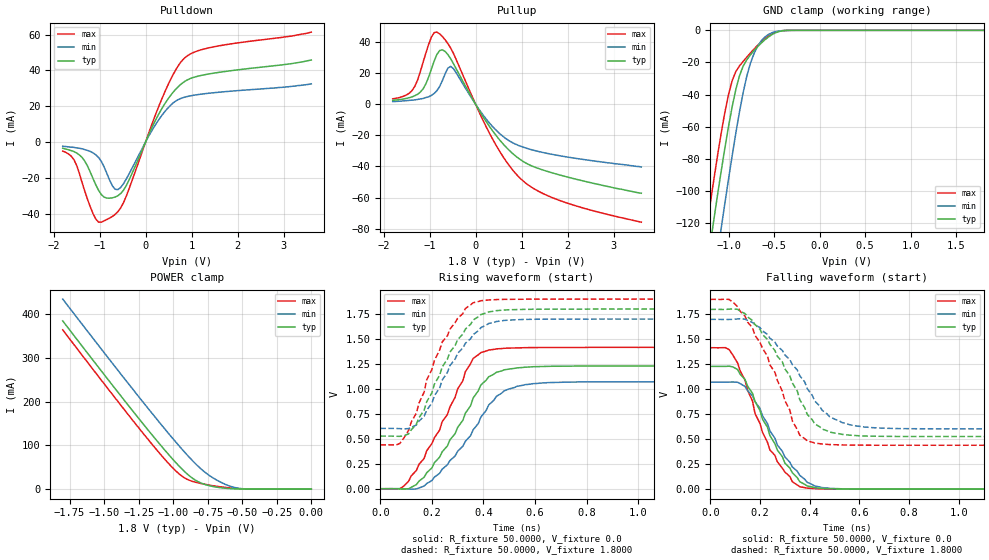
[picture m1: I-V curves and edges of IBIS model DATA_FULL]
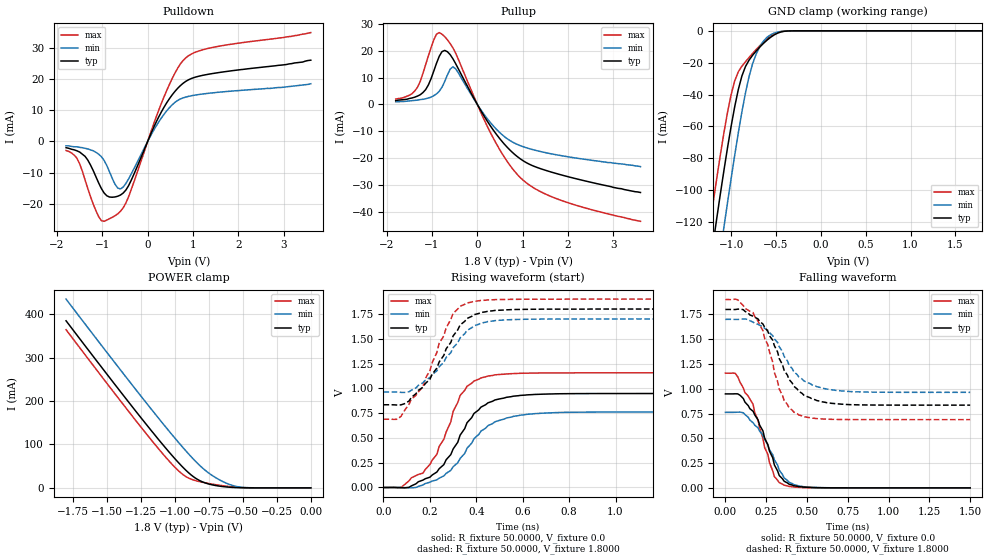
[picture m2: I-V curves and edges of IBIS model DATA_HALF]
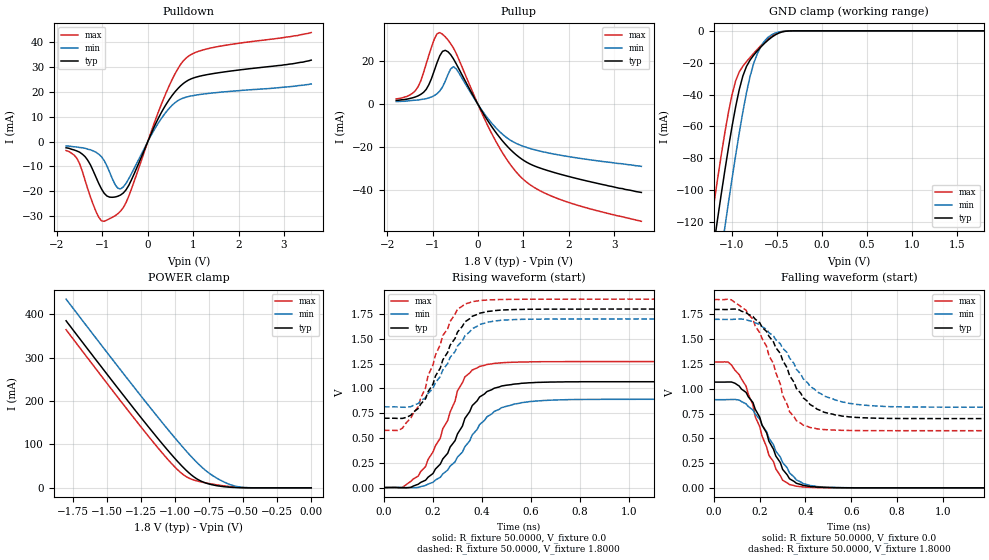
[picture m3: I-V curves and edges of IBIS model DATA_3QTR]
| IBIS file usesk1g16ai.ibs created by s2ibis3 verion 1.1
| North Carolina State University, ERL, 2006
| This Model is valid for Industrial Temperature Range -40C<=Tc<=85C
| Valid for LPDDR-333/400 operation
| Part Number   VDD/VDDQ   Package   Architecture
| SCE18K1G160AF   1.8 +0.1/-0.1  60-Ball FBGA   64Meg x 16
[IBIS Ver]   3.2
[File name]  usesk1g16ai.ibs
[File Rev]   1.2
[Date]   2015-10-27
[Source]   Simulation of a silicon level SPICE model
[Notes]   IBIS Characteristics for I/O Buffer
   IBIS Model Revision History:
Rev 1.1: 2015-10-27
   - IBIS model file initial creation
Rev 1.2: 2016-10-27
   - Updata company and other informations
[disclaimer] The IBIS models are for modeling purpose only and are
   subject to change without any notice. UniIC is not
   responsible for any problems the models may cause.
[Copyright]  Copyright 2015 UniIC Semiconductors Corp. All rights reserved
|   Component SCE18K1G160AF
[Component]   SCE18K1G160AF
[Manufacturer]  UniIC Semiconductors Corp.
| All balls excluding NC, POWER and GND (R[Ohm], L[H], C[F])
[Package]   | 60-Ball FBGA
|Variable   typ   min   max
R_pkg   366m   250m   672m
L_pkg   1.68n   1.12n   2.83n
C_pkg   0.31p   0.20p   0.55p
[Pin]   signal_name model_name   R_pin   L_pin   C_pin
A1   VSS   GND
A2   DQ15   DQ   374m   1.51n   0.32p
A3   VSSQ   GND
A7   VDDQ   POWER
A8   DQ0   DQ   390m   1.48n   0.35p
A9   VDD   POWER
B2   DQ13   DQ   444m   2n   0.4p
B3   DQ14   DQ   332m   1.35n   0.29p
B7   DQ1   DQ   268m   1.19n   0.25p
B8   DQ2   DQ   410m   1.6n   0.37p
B9   VSSQ   GND
C1   VSSQ   GND
C2   DQ11   DQ   370m   1.5n   0.34p
C3   DQ12   DQ   318m   1.58n   0.29p
C7   DQ3   DQ   294m   1.27n   0.28p
C8   DQ4   DQ   387m   1.66n   0.36p
C9   VDDQ   POWER
D1   VDDQ   POWER
D2   DQ9   DQ   391m   1.83n   0.33p
D3   DQ10   DQ   267m   1.14n   0.24p
D7   DQ5   DQ   250m   1.12n   0.27p
D8   DQ6   DQ   405m   1.87n   0.32p
D9   VSSQ   GND
E1   VSSQ   GND
E2   UDQS   DQ   406m   1.72n   0.37p
E3   DQ8   DQ   276m   1.28n   0.25p
E7   DQ7   DQ   275m   1.47n   0.21p
E8   LDQS   DQ   395m   1.59n   0.32p
E9   VDDQ   POWER
F1   VSS   GND
F2   UDM   DATA_RCV   388m   1.82n   0.32p
F7   A13   CLKCA_RCV   264m   1.18n   0.24p
F8   LDM   DATA_RCV   398m   1.54n   0.36p
F9   VDD   POWER
G1   CKE   CLKCA_RCV   453m   2.62n   0.36p
G2   CK   CLKCA_RCV   364m   1.97n   0.32p
G3   CK#   CLKCA_RCV   353m   1.72n   0.25p
G7   WE#   CLKCA_RCV   284m   1.32n   0.26p
G8   CAS#   CLKCA_RCV   381m   1.69n   0.35p
G9   RAS#   CLKCA_RCV   474m   2.32n   0.4p
H1   A9   CLKCA_RCV   457m   2.73n   0.33p
H2   A11   CLKCA_RCV   388m   2.17n   0.29p
H3   A12   CLKCA_RCV   263m   1.36n   0.25p
H7   CS#   CLKCA_RCV   262m   1.22n   0.24p
H8   BA0   CLKCA_RCV   394m   1.67n   0.36p
H9   BA1   CLKCA_RCV   508m   2.19n   0.42p
J1   A6   CLKCA_RCV   672m   2.79n   0.55p
J2   A7   CLKCA_RCV   380m   1.64n   0.3p
J3   A8   CLKCA_RCV   253m   1.34n   0.2p
J7   A10   CLKCA_RCV   263m   1.28n   0.22p
J8   A0   CLKCA_RCV   364m   1.68n   0.29p
J9   A1   CLKCA_RCV   661m   2.83n   0.54p
K1   VSS   GND
K2   A4   CLKCA_RCV   412m   1.87n   0.34p
K3   A5   CLKCA_RCV   266m   1.3n   0.23p
K7   A2   CLKCA_RCV   250m   1.18n   0.24p
K8   A3   CLKCA_RCV   367m   1.75n   0.31p
K9   VDD   POWER
|*****************************  Diff Pin  *************************************
[Diff Pin]  inv_pin  vdiff   tdelay_typ  tdelay_min  tdelay_max
G2   G3   1.08V   NA   NA   NA
|*****************************  Model Selector ********************************
[Model Selector]   DQ
DATA_FULL   Full-Strength Output Driver
DATA_3QTR   75% Strength Output Driver
DATA_HALF   Half-Strength Output Driver
DATA_RCV   Data/Data Strobe/Data Mask Receiver
| Models and submodels in the file (5): DATA_FULL (I/O), DATA_HALF (I/O), DATA_3QTR (I/O), DATA_RCV (Input), CLKCA_RCV (Input)
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|   Model DATA_FULL
[Model]  DATA_FULL
Model_type   I/O
Polarity   Non-Inverting
Enable   Active-High
Vinl  = 360.000mV
Vinh  = 1440.000mV
Vmeas = 900.000mV
Cref  = 20.000pF
C_comp   2.0990pF   2.0750pF   2.3110pF
[Temperature Range]   25.0000   85.0000   -40.0000
[Voltage Range]   1.8000V   1.7000V   1.9000V
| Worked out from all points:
|   slope of the pulldown table from 0 to 0.27 V, typ, clamps not added: 18.2 ohm
|   slope of the pullup table from 0 to 0.27 V, typ, clamps not added: 21 ohm
|   GND clamp passes 1 mA (typ) near -0.46 V on its own axis
|   POWER clamp passes 1 mA (typ) near -0.57 V on its own axis
|   rising waveform, R_fixture 50.0000, V_fixture 0.0: 20-80 % time 173ps typ, 179ps min, 163ps max; typ from 0 V to 1.23 V
|   rising waveform, R_fixture 50.0000, V_fixture 1.8000: 20-80 % time 150ps typ, 150ps min, 139ps max; typ from 0.527 V to 1.8 V
|   falling waveform, R_fixture 50.0000, V_fixture 0.0: 20-80 % time 143ps typ, 148ps min, 137ps max; typ from 1.23 V to 0 V
|   falling waveform, R_fixture 50.0000, V_fixture 1.8000: 20-80 % time 174ps typ, 187ps min, 155ps max; typ from 1.8 V to 0.527 V
[Pulldown]
|Voltage   I(typ)   I(min)   I(max)
-1.8V     -3.5mA     -2.4mA     -5.1mA
-1.56V    -5.3mA     -3mA       -9.7mA
-1.38V    -8.6mA     -3.8mA     -22.6mA
-1.14V    -20.5mA    -6.1mA     -40.14mA
-960mV    -29.42mA   -10.9mA    -44.81mA
-720mV    -31.19mA   -24.52mA   -41.6mA
-600mV    -29.99mA   -26.62mA   -38.88mA
-420mV    -24.42mA   -20.73mA   -30.32mA
300mV     16.25mA    12.96mA    20.78mA
840mV     33.67mA    24.97mA    46.74mA
1.44V     38.29mA    27.41mA    52.96mA
3.6V      45.8mA     32.5mA     61.4mA
[Pullup]
|Voltage   I(typ)   I(min)   I(max)
-1.8V     2.5mA      1.7mA      3.5mA
-1.38V    4.7mA      2.6mA      8.8mA
-1.26V    6.4mA      3.1mA      15.5mA
-1.14V    9.9mA      3.7mA      26.99mA
-960mV    22.59mA    5.67mA     43.09mA
-840mV    31.99mA    8.72mA     46.37mA
-720mV    34.94mA    15.29mA    43.47mA
-540mV    29.17mA    24.33mA    36.08mA
300mV     -14.19mA   -12.02mA   -18.52mA
960mV     -35.32mA   -26.79mA   -47.34mA
1.86V     -45.72mA   -33.27mA   -62.2mA
3.6V      -57.2mA    -40.3mA    -75.8mA
[GND_clamp]
|Voltage   I(typ)   I(min)   I(max)
-1.8V     -382.1mA   -420.9mA   -357.5mA
-1.24V    -149mA     -187mA     -123.6mA
-1.16V    -117.7mA   -154.8mA   -92.62mA
-1.08V    -87.61mA   -123.2mA   -63.92mA
-1V       -59.95mA   -92.78mA   -40.06mA
-960mV    -47.64mA   -78.15mA   -31.42mA
-880mV    -28.39mA   -50.93mA   -22.22mA
-800mV    -18.4mA    -28.71mA   -16.75mA
-680mV    -10.16mA   -9.871mA   -9.318mA
-560mV    -4.068mA   -2.483mA   -3.393mA
-360mV    -77.71uA   -65.53uA   -56.11uA
1.8V      3.312nA    24.23nA    479.4pA
[POWER_clamp]
|Voltage   I(typ)   I(min)   I(max)
-1.8V     384.7mA    434.6mA    364.2mA
-1.38V    213.6mA    263.5mA    192.2mA
-1.16V    126.8mA    176.1mA    105.2mA
-1.02V    74.41mA    122.2mA    54.12mA
-960mV    53.65mA    99.93mA    35.62mA
-920mV    40.93mA    85.55mA    26.2mA
-840mV    20.7mA     58.65mA    16mA
-780mV    11.76mA    41.29mA    11.75mA
-680mV    4.343mA    19.92mA    6.353mA
-580mV    1.115mA    5.926mA    2.488mA
-460mV    97.61uA    425uA      237.2uA
0V        3.312nA    8.237nA    602.9pA
[Ramp]
| variable   typ   min   max
dV/dt_r  0.7374/0.1699n   0.6426/0.1795n   0.8496/0.1636n
dV/dt_f  0.7638/0.1717n   0.6576/0.1866n   0.8762/0.1570n
R_load = 50.0000
[Rising Waveform]
R_fixture= 50.0000
V_fixture= 0.0
V_fixture_min= 0.0
V_fixture_max= 0.0
|time   V(typ)   V(min)   V(max)
0s        0V         0V         0V
90.91ps   -4.216mV   -497.2uV   25.92mV
170ps     115mV      26.85mV    303.9mV
260ps     428mV      239.4mV    743.1mV
330ps     757mV      475.9mV    1.173V
360ps     908.9mV    590.6mV    1.306V
390ps     1.04V      719.2mV    1.364V
480ps     1.191V     980.7mV    1.407V
590ps     1.222V     1.052V     1.414V
1.5ns     1.229V     1.071V     1.416V
[Rising Waveform]
R_fixture= 50.0000
V_fixture= 1.8000
V_fixture_min= 1.7000
V_fixture_max= 1.9000
|time   V(typ)   V(min)   V(max)
0s        527mV      604mV      439.6mV
75.76ps   524.6mV    601.8mV    452.9mV
140ps     646.7mV    638.8mV    758.4mV
180ps     871.9mV    786.2mV    1.091V
200ps     959.8mV    857mV      1.194V
240ps     1.22V      1.089V     1.47V
360ps     1.69V      1.544V     1.863V
420ps     1.771V     1.655V     1.891V
520ps     1.794V     1.692V     1.898V
1.5ns     1.8V       1.7V       1.9V
[Falling Waveform]
R_fixture= 50.0000
V_fixture= 0.0
V_fixture_min= 0.0
V_fixture_max= 0.0
|time   V(typ)   V(min)   V(max)
0s        1.229V     1.071V     1.416V
75.76ps   1.231V     1.072V     1.397V
110ps     1.197V     1.07V      1.262V
170ps     959.1mV    934.7mV    880.3mV
180ps     877.9mV    875.6mV    757.3mV
240ps     535.2mV    582.8mV    392.4mV
300ps     261.6mV    322.9mV    171.5mV
360ps     74.58mV    138.3mV    24.6mV
480ps     4.177mV    8.446mV    1.502mV
1.5ns     0V         -795nV     0V
[Falling Waveform]
R_fixture= 50.0000
V_fixture= 1.8000
V_fixture_min= 1.7000
V_fixture_max= 1.9000
|time   V(typ)   V(min)   V(max)
0s        1.8V       1.7V       1.9V
75.76ps   1.802V     1.699V     1.899V
170ps     1.688V     1.669V     1.615V
260ps     1.388V     1.472V     1.17V
330ps     1.063V     1.247V     684.1mV
360ps     894.7mV    1.136V     540.1mV
390ps     748.2mV    1.006V     483.8mV
480ps     571.5mV    724.7mV    446.4mV
590ps     535.5mV    631.1mV    440.6mV
1.5ns     527mV      604mV      439.6mV
|   Model DATA_HALF
[Model]  DATA_HALF
Model_type   I/O
Polarity   Non-Inverting
Enable   Active-High
Vinl  = 360.000mV
Vinh  = 1440.000mV
Vmeas = 900.000mV
Cref  = 20.000pF
C_comp   2.0990pF   2.0750pF   2.3110pF
[Temperature Range]   25.0000   85.0000   -40.0000
[Voltage Range]   1.8000V   1.7000V   1.9000V
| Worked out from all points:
|   slope of the pulldown table from 0 to 0.27 V, typ, clamps not added: 31.3 ohm
|   slope of the pullup table from 0 to 0.27 V, typ, clamps not added: 36.1 ohm
|   GND clamp passes 1 mA (typ) near -0.46 V on its own axis
|   POWER clamp passes 1 mA (typ) near -0.57 V on its own axis
|   rising waveform, R_fixture 50.0000, V_fixture 0.0: 20-80 % time 156ps typ, 168ps min, 130ps max; typ from 0 V to 0.948 V
|   rising waveform, R_fixture 50.0000, V_fixture 1.8000: 20-80 % time 149ps typ, 150ps min, 141ps max; typ from 0.834 V to 1.8 V
|   falling waveform, R_fixture 50.0000, V_fixture 0.0: 20-80 % time 140ps typ, 145ps min, 136ps max; typ from 0.948 V to 0 V
|   falling waveform, R_fixture 50.0000, V_fixture 1.8000: 20-80 % time 172ps typ, 179ps min, 144ps max; typ from 1.8 V to 0.834 V
[Pulldown]
|Voltage   I(typ)   I(min)   I(max)
-1.8V     -2mA       -1.4mA     -2.9mA
-1.56V    -3mA       -1.7mA     -5.4mA
-1.38V    -4.8mA     -2.2mA     -12.4mA
-1.08V    -13.39mA   -4.1mA     -24.25mA
-900mV    -17.51mA   -7.78mA    -25.32mA
-660mV    -17.64mA   -15.01mA   -23.33mA
-540mV    -16.62mA   -14.68mA   -21.38mA
300mV     9.454mA    7.512mA    12.17mA
600mV     16.1mA     12.58mA    21.97mA
840mV     19.36mA    14.31mA    26.95mA
1.5V      22.05mA    15.77mA    30.5mA
3.6V      26.2mA     18.6mA     35.1mA
[Pullup]
|Voltage   I(typ)   I(min)   I(max)
-1.8V     1.4mA      1mA        2mA
-1.32V    3.1mA      1.6mA      6.4mA
-1.08V    7.23mA     2.4mA      18.01mA
-960mV    12.42mA    3.27mA     23.99mA
-840mV    17.87mA    4.9mA      26.69mA
-720mV    20.06mA    8.48mA     25.18mA
-540mV    17mA       13.97mA    21.07mA
300mV     -8.245mA   -6.961mA   -10.82mA
660mV     -15.91mA   -12.74mA   -21.2mA
960mV     -20.34mA   -15.38mA   -27.35mA
1.86V     -26.2mA    -19.05mA   -35.69mA
3.6V      -32.7mA    -23.1mA    -43.4mA
[GND_clamp]
|Voltage   I(typ)   I(min)   I(max)
-1.8V     -382.1mA   -420.9mA   -357.5mA
-1.24V    -149mA     -187mA     -123.6mA
-1.16V    -117.7mA   -154.8mA   -92.62mA
-1.08V    -87.61mA   -123.2mA   -63.92mA
-1V       -59.95mA   -92.78mA   -40.06mA
-960mV    -47.64mA   -78.15mA   -31.42mA
-880mV    -28.39mA   -50.93mA   -22.22mA
-800mV    -18.4mA    -28.71mA   -16.75mA
-680mV    -10.16mA   -9.871mA   -9.318mA
-560mV    -4.068mA   -2.483mA   -3.393mA
-360mV    -77.71uA   -65.53uA   -56.11uA
1.8V      3.312nA    24.23nA    479.4pA
[POWER_clamp]
|Voltage   I(typ)   I(min)   I(max)
-1.8V     384.7mA    434.6mA    364.2mA
-1.38V    213.6mA    263.5mA    192.2mA
-1.16V    126.8mA    176.1mA    105.2mA
-1.02V    74.41mA    122.2mA    54.12mA
-960mV    53.65mA    99.93mA    35.62mA
-920mV    40.93mA    85.55mA    26.2mA
-840mV    20.7mA     58.65mA    16mA
-780mV    11.76mA    41.29mA    11.75mA
-680mV    4.343mA    19.92mA    6.353mA
-580mV    1.115mA    5.926mA    2.488mA
-460mV    97.61uA    425uA      237.2uA
0V        3.312nA    8.237nA    602.9pA
[Ramp]
| variable   typ   min   max
dV/dt_r  0.5687/0.1549n   0.4570/0.1668n   0.6942/0.1347n
dV/dt_f  0.5793/0.1729n   0.4419/0.1794n   0.7270/0.1406n
R_load = 50.0000
[Rising Waveform]
R_fixture= 50.0000
V_fixture= 0.0
V_fixture_min= 0.0
V_fixture_max= 0.0
|time   V(typ)   V(min)   V(max)
0s        0V         0V         0V
75.76ps   -2.229mV   491.3uV    1.445mV
170ps     74.53mV    25.4mV     144.2mV
230ps     155.9mV    77.15mV    334.3mV
290ps     331.8mV    173mV      661.6mV
330ps     527.3mV    292.8mV    927.6mV
420ps     811mV      568.5mV    1.105V
530ps     909.9mV    701mV      1.145V
650ps     938.4mV    744.7mV    1.154V
1.5ns     947.9mV    761.7mV    1.157V
[Rising Waveform]
R_fixture= 50.0000
V_fixture= 1.8000
V_fixture_min= 1.7000
V_fixture_max= 1.9000
|time   V(typ)   V(min)   V(max)
0s        834.5mV    963.5mV    688.4mV
60.61ps   831.5mV    962.1mV    688.5mV
110ps     872mV      965.5mV    839.2mV
170ps     1.011V     1.056V     1.017V
230ps     1.204V     1.176V     1.362V
240ps     1.267V     1.218V     1.455V
300ps     1.529V     1.41V      1.757V
360ps     1.705V     1.585V     1.861V
530ps     1.792V     1.691V     1.897V
1.5ns     1.8V       1.7V       1.9V
[Falling Waveform]
R_fixture= 50.0000
V_fixture= 0.0
V_fixture_min= 0.0
V_fixture_max= 0.0
|time   V(typ)   V(min)   V(max)
0s        947.9mV    761.7mV    1.157V
60.61ps   948.9mV    762.2mV    1.155V
110ps     900.9mV    757mV      1.007V
170ps     772.5mV    656.6mV    841mV
230ps     574.9mV    532.6mV    499mV
240ps     505.7mV    488.2mV    408.3mV
300ps     232mV      282.8mV    114.3mV
360ps     67.03mV    100.4mV    26.74mV
530ps     3.545mV    5.524mV    1.264mV
1.5ns     0V         0V         0V
[Falling Waveform]
R_fixture= 50.0000
V_fixture= 1.8000
V_fixture_min= 1.7000
V_fixture_max= 1.9000
|time   V(typ)   V(min)   V(max)
0s        1.8V       1.7V       1.9V
75.76ps   1.803V     1.699V     1.897V
170ps     1.732V     1.672V     1.767V
260ps     1.58V      1.59V      1.444V
330ps     1.304V     1.424V     996mV
360ps     1.186V     1.326V     881.5mV
450ps     973.6mV    1.119V     735.4mV
560ps     880.9mV    1.021V     698.5mV
710ps     844.3mV    978mV      689.7mV
1.5ns     834.5mV    963.5mV    688.4mV
|   Model DATA_3QTR
[Model]  DATA_3QTR
Model_type   I/O
Polarity   Non-Inverting
Enable   Active-High
Vinl  = 360.000mV
Vinh  = 1440.000mV
Vmeas = 900.000mV
Cref  = 20.000pF
C_comp   2.0990pF   2.0750pF   2.3110pF
[Temperature Range]   25.0000   85.0000   -40.0000
[Voltage Range]   1.8000V   1.7000V   1.9000V
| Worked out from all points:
|   slope of the pulldown table from 0 to 0.27 V, typ, clamps not added: 25.2 ohm
|   slope of the pullup table from 0 to 0.27 V, typ, clamps not added: 29 ohm
|   GND clamp passes 1 mA (typ) near -0.46 V on its own axis
|   POWER clamp passes 1 mA (typ) near -0.57 V on its own axis
|   rising waveform, R_fixture 50.0000, V_fixture 0.0: 20-80 % time 151ps typ, 159ps min, 134ps max; typ from 0 V to 1.07 V
|   rising waveform, R_fixture 50.0000, V_fixture 1.8000: 20-80 % time 131ps typ, 132ps min, 122ps max; typ from 0.699 V to 1.8 V
|   falling waveform, R_fixture 50.0000, V_fixture 0.0: 20-80 % time 125ps typ, 132ps min, 120ps max; typ from 1.07 V to 0 V
|   falling waveform, R_fixture 50.0000, V_fixture 1.8000: 20-80 % time 159ps typ, 179ps min, 140ps max; typ from 1.8 V to 0.699 V
[Pulldown]
|Voltage   I(typ)   I(min)   I(max)
-1.8V     -2.5mA     -1.8mA     -3.6mA
-1.56V    -3.8mA     -2.2mA     -6.8mA
-1.38V    -6.1mA     -2.7mA     -15.7mA
-1.08V    -16.89mA   -5.1mA     -30.48mA
-900mV    -21.93mA   -9.81mA    -31.6mA
-660mV    -22.02mA   -18.8mA    -29.07mA
-540mV    -20.71mA   -18.28mA   -26.57mA
300mV     11.75mA    9.345mA    15.09mA
600mV     20.05mA    15.68mA    27.29mA
840mV     24.15mA    17.87mA    33.59mA
1.44V     27.38mA    19.6mA     37.88mA
3.6V      32.8mA     23.2mA     43.9mA
[Pullup]
|Voltage   I(typ)   I(min)   I(max)
-1.8V     1.8mA      1.3mA      2.5mA
-1.5V     2.7mA      1.7mA      4.3mA
-1.32V    3.9mA      2mA        8.1mA
-1.08V    9.13mA     3mA        22.84mA
-960mV    15.72mA    4.07mA     30.26mA
-840mV    22.51mA    6.16mA     33.29mA
-720mV    25.04mA    10.7mA     31.33mA
-540mV    21.11mA    17.44mA    26.15mA
360mV     -12.05mA   -10.11mA   -15.83mA
960mV     -25.36mA   -19.19mA   -34.06mA
1.8V      -32.38mA   -23.57mA   -44.09mA
3.6V      -40.9mA    -28.8mA    -54.3mA
[GND_clamp]
|Voltage   I(typ)   I(min)   I(max)
-1.8V     -382.1mA   -420.9mA   -357.5mA
-1.24V    -149mA     -187mA     -123.6mA
-1.16V    -117.7mA   -154.8mA   -92.62mA
-1.08V    -87.61mA   -123.2mA   -63.92mA
-1V       -59.95mA   -92.78mA   -40.06mA
-960mV    -47.64mA   -78.15mA   -31.42mA
-880mV    -28.39mA   -50.93mA   -22.22mA
-800mV    -18.4mA    -28.71mA   -16.75mA
-680mV    -10.16mA   -9.871mA   -9.318mA
-560mV    -4.068mA   -2.483mA   -3.393mA
-360mV    -77.71uA   -65.53uA   -56.11uA
1.8V      3.312nA    24.23nA    479.4pA
[POWER_clamp]
|Voltage   I(typ)   I(min)   I(max)
-1.8V     384.7mA    434.6mA    364.2mA
-1.38V    213.6mA    263.5mA    192.2mA
-1.16V    126.8mA    176.1mA    105.2mA
-1.02V    74.41mA    122.2mA    54.12mA
-960mV    53.65mA    99.93mA    35.62mA
-920mV    40.93mA    85.55mA    26.2mA
-840mV    20.7mA     58.65mA    16mA
-780mV    11.76mA    41.29mA    11.75mA
-680mV    4.343mA    19.92mA    6.353mA
-580mV    1.115mA    5.926mA    2.488mA
-460mV    97.61uA    425uA      237.2uA
0V        3.312nA    8.237nA    602.9pA
[Ramp]
| variable   typ   min   max
dV/dt_r  0.6402/0.1506n   0.5339/0.1638n   0.7620/0.1338n
dV/dt_f  0.6607/0.1623n   0.5318/0.1784n   0.7940/0.1355n
R_load = 50.0000
[Rising Waveform]
R_fixture= 50.0000
V_fixture= 0.0
V_fixture_min= 0.0
V_fixture_max= 0.0
|time   V(typ)   V(min)   V(max)
0s        0V         0V         0V
75.76ps   -2.198mV   433.8uV    1.666mV
140ps     33.44mV    628.7uV    116mV
200ps     141.5mV    52.45mV    358.2mV
290ps     472.6mV    259.4mV    872mV
330ps     696.5mV    411.5mV    1.115V
390ps     913mV      634.7mV    1.221V
480ps     1.024V     805.5mV    1.258V
620ps     1.06V      872.7mV    1.268V
1.5ns     1.067V     889.9mV    1.27V
[Rising Waveform]
R_fixture= 50.0000
V_fixture= 1.8000
V_fixture_min= 1.7000
V_fixture_max= 1.9000
|time   V(typ)   V(min)   V(max)
0s        698.8mV    813.6mV    576.6mV
75.76ps   697.5mV    809.8mV    599.9mV
140ps     797.7mV    847.7mV    816.2mV
200ps     1.042V     1V         1.236V
240ps     1.287V     1.186V     1.533V
300ps     1.568V     1.427V     1.798V
330ps     1.67V      1.529V     1.851V
390ps     1.758V     1.644V     1.886V
480ps     1.79V      1.688V     1.896V
1.5ns     1.8V       1.7V       1.9V
[Falling Waveform]
R_fixture= 50.0000
V_fixture= 0.0
V_fixture_min= 0.0
V_fixture_max= 0.0
|time   V(typ)   V(min)   V(max)
0s        1.067V     889.9mV    1.27V
60.61ps   1.068V     890.3mV    1.27V
140ps     963.2mV    847.2mV    1.026V
200ps     711.8mV    692.2mV    616.2mV
240ps     470mV      500.9mV    327.5mV
300ps     186.4mV    255.6mV    77.44mV
330ps     92.05mV    151mV      33.55mV
390ps     24.43mV    42.73mV    8.693mV
480ps     4.545mV    7.823mV    1.617mV
1.5ns     0V         0V         0V
[Falling Waveform]
R_fixture= 50.0000
V_fixture= 1.8000
V_fixture_min= 1.7000
V_fixture_max= 1.9000
|time   V(typ)   V(min)   V(max)
0s        1.8V       1.7V       1.9V
75.76ps   1.803V     1.699V     1.897V
170ps     1.729V     1.677V     1.703V
260ps     1.472V     1.532V     1.253V
300ps     1.287V     1.409V     934mV
330ps     1.134V     1.311V     769.3mV
390ps     908.1mV    1.1V       632.4mV
480ps     763.7mV    927.7mV    588.1mV
620ps     710.8mV    842.8mV    578mV
1.5ns     698.8mV    813.6mV    576.6mV
